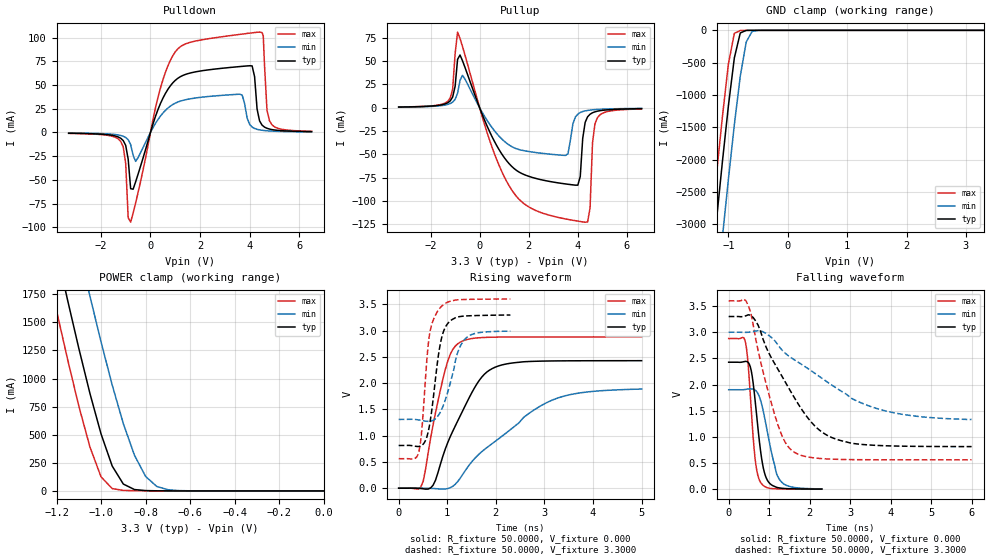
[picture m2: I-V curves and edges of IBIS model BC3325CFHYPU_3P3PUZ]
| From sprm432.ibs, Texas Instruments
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|   Model BC3325CFHYPU_3P3PUZ
[Model]   BC3325CFHYPU_3P3PUZ
Model_type   I/O
Polarity   Non-Inverting
Enable   Active-Low
Vinl =   0.9900V
Vinh =   2.3100V
Vmeas =   1.6500V
Cref =  15.0000pF
Rref = 100.0000M
Vref =  0.000V
C_comp   3.2113000062pf   3.3653001534pf   5.2276998132pf
[Temperature Range]   25.0000   0.1250k   -40.0000
[Voltage Range]   3.3000V   3.0000V   3.6000V
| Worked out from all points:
|   slope of the pulldown table from 0 to 0.495 V, typ, clamps not added: 13.9 ohm
|   slope of the pullup table from 0 to 0.495 V, typ, clamps not added: 16.3 ohm
|   GND clamp passes 1 mA (typ) near -0.68 V on its own axis
|   POWER clamp passes 1 mA (typ) near -0.74 V on its own axis
|   rising waveform, R_fixture 50.0000, V_fixture 0.000: 20-80 % time 713ps typ, 1.42ns min, 383ps max; typ from 0 V to 2.43 V
|   rising waveform, R_fixture 50.0000, V_fixture 3.3000: 20-80 % time 215ps typ, 298ps min, 166ps max; typ from 0.814 V to 3.29 V
|   falling waveform, R_fixture 50.0000, V_fixture 0.000: 20-80 % time 217ps typ, 310ps min, 165ps max; typ from 2.43 V to 0.003 V
|   falling waveform, R_fixture 50.0000, V_fixture 3.3000: 20-80 % time 1.13ns typ, 1.92ns min, 604ps max; typ from 3.3 V to 0.814 V
[Pulldown]
| voltage   I(typ)   I(min)   I(max)
-3.3V     -858uA     -614uA     -1.004mA
-1.2V     -6.162mA   -3.225mA   -9.461mA
-800mV    -59.28mA   -12.78mA   -94.65mA
-600mV    -52.16mA   -30.51mA   -74.44mA
1V        54.91mA    30.86mA    84.97mA
3.6V      69.44mA    40.27mA    103.4mA
4.1V      70.14mA    5.645mA    105mA
4.4V      12.22mA    2.696mA    105.8mA
4.55V     6.668mA    2.131mA    101.9mA
4.7V      4.353mA    1.744mA    23.59mA
4.8V      3.553mA    1.558mA    12.25mA
6.5V      840uA      548uA      1.177mA
|   6.6000   0.8040mA   0.5280mA   1.1170mA
[Pullup]
| voltage   I(typ)   I(min)   I(max)
-3.3V     804uA      687uA      859uA
-1.3V     5.391mA    3.609mA    6.959mA
-900mV    51.9mA     15.62mA    81.15mA
600mV     -35.88mA   -24.51mA   -49.07mA
1.7V      -70.21mA   -45.37mA   -100.4mA
3.5V      -81.59mA   -51.02mA   -119.1mA
4V        -82.9mA    -6.76mA    -121.4mA
4.3V      -15.54mA   -3.316mA   -122.6mA
4.5V      -6.855mA   -2.452mA   -107.1mA
4.6V      -5.293mA   -2.167mA   -37.39mA
4.8V      -3.613mA   -1.755mA   -10.57mA
6.6V      -914uA     -641uA     -1.25mA
[GND_clamp]
| voltage   I(typ)   I(min)   I(max)
-3.3V     -23.4A     -24.49A    -22.76A
-1.3V     -3.859A    -5.036A    -3.154A
-1.2V     -2.93A     -4.106A    -2.224A
-1.1V     -2.025A    -3.192A    -1.329A
-1V       -1.167A    -2.304A    -520.4mA
-900mV    -427mA     -1.461A    -46.26mA
-800mV    -40.87mA   -709.2mA   -2.663mA
-700mV    -1.282mA   -180.3mA   -248.5uA
-600mV    -50.08uA   -16.03mA   -13.99uA
-400mV    -107.5nA   -55.51uA   -12.38nA
3.3V      288pA      878nA      263.1pA
[POWER_clamp]
| voltage   I(typ)   I(min)   I(max)
-3.3V     22.53A     23.34A     22.08A
-1.25V    2.586A     3.492A     2.054A
-1.2V     2.135A     3.04A      1.604A
-1.15V    1.695A     2.594A     1.168A
-1.05V    867.5mA    1.733A     390.4mA
-1V       506.6mA    1.325A     124.9mA
-950mV    221.4mA    942.3mA    20.91mA
-900mV    61.12mA    598.6mA    4.55mA
-850mV    12.31mA    317.4mA    2.13mA
-800mV    3.023mA    129mA      1.192mA
-750mV    1.142mA    39.95mA    599.5uA
0V        288pA      1.9nA      334.1pA
[Ramp]
| variable   typ   min   max
dV/dt_r   1.4558/0.7057n   1.1319/1.4536n   1.7275/0.3797n
dV/dt_f   1.4900/1.1147n   0.9787/1.8842n   1.8228/0.5983n
R_load = 50.0000
[Rising Waveform]
R_fixture = 50.0000
V_fixture = 0.000
V_fixture_min = 0.000
V_fixture_max = 0.000
| time   V(typ)   V(min)   V(max)
0s        1.169nV    5.523nV    878.9pV
454.5ps   -5.613mV   1.471mV    21.26mV
505.1ps   -11.27mV   1.254mV    133.5mV
707.1ps   55.83mV    -4.995mV   1.2V
959.6ps   746.1mV    -14.74mV   2.258V
1.263ns   1.369V     185.4mV    2.777V
1.667ns   2.062V     659.3mV    2.863V
2.071ns   2.331V     950.2mV    2.875V
3.283ns   2.423V     1.719V     2.879V
5ns       2.426V     1.887V     2.879V
[Rising Waveform]
R_fixture = 50.0000
V_fixture = 3.3000
V_fixture_min = 3.0000
V_fixture_max = 3.6000
| time   V(typ)   V(min)   V(max)
0s        813.5mV    1.309V     562mV
418.2ps   795.3mV    1.298V     703.1mV
487.9ps   823.6mV    1.286V     1.234V
580.8ps   977.5mV    1.273V     2.457V
627.3ps   1.159V     1.273V     2.879V
813.1ps   2.499V     1.38V      3.384V
975.8ps   3.088V     1.724V     3.525V
1.185ns   3.251V     2.499V     3.582V
1.347ns   3.275V     2.819V     3.59V
2.3ns     3.295V     2.988V     3.599V
[Falling Waveform]
R_fixture = 50.0000
V_fixture = 0.000
V_fixture_min = 0.000
V_fixture_max = 0.000
| time   V(typ)   V(min)   V(max)
0s        2.427V     1.901V     2.879V
418.2ps   2.443V     1.907V     2.794V
464.6ps   2.434V     1.913V     2.528V
534.3ps   2.339V     1.918V     1.8V
650.5ps   1.716V     1.895V     598.7mV
789.9ps   718.3mV    1.694V     129.1mV
952.5ps   176.3mV    1.109V     29.16mV
1.185ns   35.42mV    290.2mV    7.377mV
1.254ns   24.53mV    186.2mV    6.134mV
2.3ns     2.579mV    6.474mV    824uV
[Falling Waveform]
R_fixture = 50.0000
V_fixture = 3.3000
V_fixture_min = 3.0000
V_fixture_max = 3.6000
| time   V(typ)   V(min)   V(max)
0s        3.3V       3V         3.6V
484.8ps   3.333V     2.999V     3.507V
727.3ps   3.135V     3.029V     2.646V
1.152ns   2.379V     2.826V     1.387V
1.394ns   2.054V     2.601V     899.2mV
1.636ns   1.731V     2.466V     699.7mV
2.182ns   1.169V     2.186V     592.4mV
2.788ns   925.5mV    1.87V      569mV
4ns       827.4mV    1.473V     562.4mV
6ns       814.4mV    1.332V     562mV
